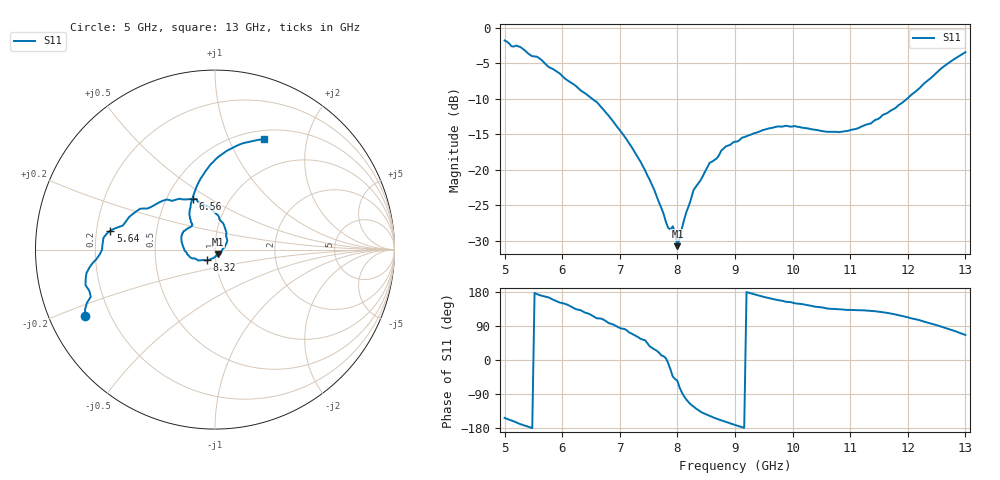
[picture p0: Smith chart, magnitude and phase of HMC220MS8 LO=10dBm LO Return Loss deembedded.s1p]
!Hittite Microwave Corporation
!12 Elizabeth Drive
!Chelmsford, MA 01824
!Tel: 978-250-3343
!Fax: 978-250-3373
!Device: HMC220MS8, 5-12 GHz, GaAS MMIC SMT Double-Balanced Mixer in 8-lead MSOP package
!Misc: LO power level=10dBm, Room
# MHZ S MA R 50
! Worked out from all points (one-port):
!   201 points, 5 GHz to 13 GHz, reference 50 ohm
!   lowest |S11| = -30.8 dB at 8 GHz (marker M1), VSWR 1.06, Z = 51.6 - j2.46 ohm
!   |S11| at or under -10 dB: 6.519 GHz to 11.99 GHz (5.47 GHz wide, 59.1 % of centre)
!   S11 on the Smith chart (normalised r, x): 5 GHz: 0.11, -0.24; 5.64 GHz: 0.26, +0.08; 6.56 GHz: 0.68, +0.42; 8.32 GHz: 0.90, -0.11; 13 GHz: 0.60, +1.35
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5000  0.813 -152.8
5120  0.74 -159.2
5280  0.728 -169.6
5640  0.593 169.7
6000  0.458 150.0
6240  0.388 134.1
6560  0.307 113.7
7000  0.19 84.5
7440  0.099 52.0
7600  0.072 28.0
7840  0.039 -8.2
7920  0.04 -43.8
7960  0.036 -50.1
8000  0.029 -55.0
8160  0.051 -105.2
8320  0.076 -127.8
8560  0.112 -147.3
8840  0.146 -163.2
9000  0.158 -171.4
9600  0.196 163.0
10000  0.202 151.1
10600  0.185 135.9
11000  0.19 132.2
11480  0.227 127.8
12000  0.319 112.7
12480  0.474 93.1
12760  0.585 78.9
13000  0.672 66.2
